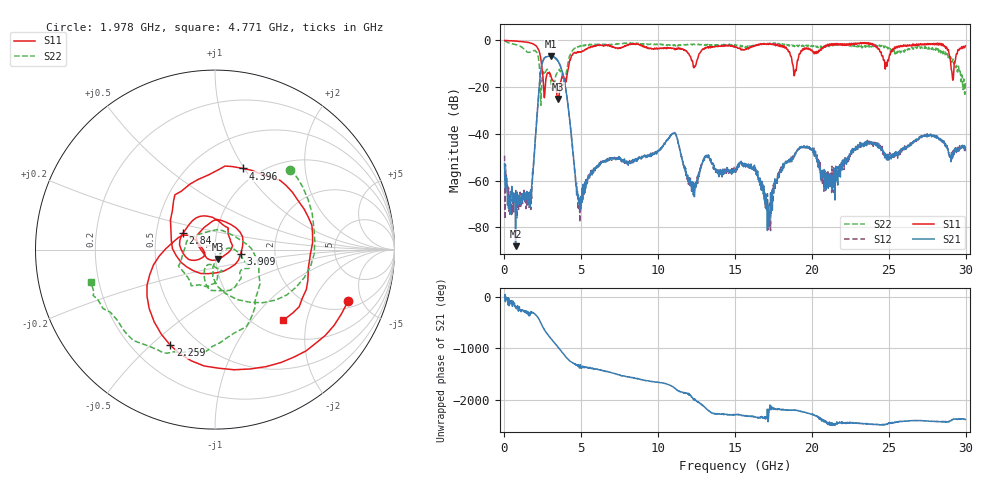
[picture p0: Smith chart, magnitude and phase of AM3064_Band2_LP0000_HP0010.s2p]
# Hz S DB R 50.0
!freq dBS11 angS11 dBS21 angS21 dBS12 angS12 dBS22 angS22
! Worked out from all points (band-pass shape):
!   1600 points, 10 MHz to 29.98 GHz, reference 50 ohm
!   highest |S21| = -6.67 dB at 3.046 GHz (marker M1); lowest = -88.0 dB at 722.3 MHz (marker M2)
!   |S21| within 3 dB of the highest: 2.459 GHz to 3.549 GHz (1.089 GHz wide, 36.3 % of centre)
!   lowest |S11| = -25.1 dB at 3.459 GHz (marker M3), VSWR 1.12, Z = 51.6 - j5.44 ohm
!   |S11| at or under -10 dB: 2.408 GHz to 4.204 GHz (1.797 GHz wide, 54.3 % of centre); 18.74 GHz to 19.02 GHz (286.8 MHz wide, 1.52 % of centre); 29.03 GHz to 29.26 GHz (228.6 MHz wide, 0.784 % of centre)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
!   |S22| runs from -27.8 to -0.2 dB; largest |S21 - S12| = 0.016
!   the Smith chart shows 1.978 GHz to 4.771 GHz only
!   S11 on the Smith chart (normalised r, x): 1.978 GHz: 2.45, -3.85; 2.259 GHz: 0.35, -0.58; 2.84 GHz: 0.69, +0.13; 3.909 GHz: 1.33, -0.07; 4.396 GHz: 0.84, +0.99; 4.771 GHz: 1.30, -1.46
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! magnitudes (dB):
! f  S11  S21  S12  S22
! 10 MHz  0.0  -52.7  -49.3  -0.2
! 722.3 MHz  -0.2  -88.0  -67.2  -1.8
! 1.641 GHz  -1.0  -71.3  -67.2  -5.1
! 1.978 GHz  -2.0  -44.7  -44.7  -4.3
! 2.259 GHz  -4.6  -20.0  -19.9  -10.3
! 2.84 GHz  -13.9  -6.8  -6.8  -12.8
! 3.046 GHz  -15.8  -6.7  -6.7  -19.0
! 3.459 GHz  -25.1  -8.6  -8.7  -13.5
! 3.909 GHz  -16.8  -17.9  -17.7  -19.0
! 4.396 GHz  -6.4  -43.9  -43.4  -4.6
! 4.771 GHz  -5.2  -66.9  -69.2  -2.9
! 5.015 GHz  -4.9  -67.7  -66.4  -2.6
! 10 GHz  -3.5  -47.2  -47.1  -1.7
! 11.09 GHz  -3.8  -39.9  -39.7  -1.9
! 12.31 GHz  -11.5  -63.7  -63.7  -1.6
! 13.13 GHz  -3.2  -49.2  -49.5  -2.0
! 15 GHz  -2.5  -55.3  -55.3  -1.9
! 17.2 GHz  -1.5  -79.6  -71.9  -1.6
! 19.99 GHz  -4.1  -46.8  -46.4  -2.2
! 20.97 GHz  -2.4  -58.5  -56.5  -2.5
! 25 GHz  -8.0  -51.1  -49.6  -3.1
! 29.98 GHz  -2.3  -47.0  -46.6  -17.4
